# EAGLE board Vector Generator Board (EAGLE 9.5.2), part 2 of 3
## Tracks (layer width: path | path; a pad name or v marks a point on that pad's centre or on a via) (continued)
DX2 (continued)
  Bottom 0.381: 3A.6 77.67,269.48 81.18,272.99 93.15,272.99 96.95,269.19 98.7,269.19 99.58,270.07 99.58,275.32 97.83,275.32 4A.3
DX3
  Bottom 0.381: 4A.4 97.54,273.28 90.23,280.58 78.84,280.58 77.67,279.41 3A.2
DX4
  Bottom 0.381: 4A.5 97.54,270.65 89.06,279.12 85.27,279.12 3A.15
DX5  (via drill 0.35)
  Top 0.381: v87.02,243.19 87.02,230.63 85.27,228.88 3B.9
  Bottom 0.381: v87.02,243.19 87.31,242.9 97.24,242.9 97.54,242.61 4B.2
DX6
  Bottom 0.381: 3B.6 77.67,233.84 78.26,234.43 80.89,234.43 83.81,237.35 93.15,237.35 96.66,233.84 99,233.84 100.17,235.01 100.17,239.98 97.83,239.98 4B.3
DX7
  Bottom 0.381: 3B.2 77.67,243.78 81.47,239.98 92.28,239.98 94.62,237.64 97.54,237.64 4B.4
DX8
  Bottom 0.381: 4B.5 97.83,235.01 99.58,236.77 99.58,238.81 94.32,238.81 90.82,242.32 86.73,242.32 85.27,243.78 3B.15
DX9  (via drill 0.35)
  Top 0.381: v89.65,207.26 v89.65,193.24
  Bottom 0.381: v89.65,193.24 85.27,193.24 3C.9 | v89.65,207.26 97.54,207.26 4C.2
DX10  (via drill 0.35)
  Top 0.381: v90.23,191.49 94.03,195.29 94.03,202.01 96.37,204.34 97.54,204.34 4C.3
  Bottom 0.381: 3C.6 84.1,191.49 v90.23,191.49
DX11  (via drill 0.35)
  Top 0.381: v95.78,199.96 97.54,201.71 4C.4
  Bottom 0.381: v95.78,199.96 91.11,204.63 83.81,204.63 80.89,207.56 78.26,207.56 77.67,208.14 3C.2
DX12
  Bottom 0.381: 4C.5 97.54,199.67 91.4,205.8 87.61,205.8 85.27,208.14 3C.15
DY1
  Top 0.381: 3D.9 85.27,157.61 89.06,157.61 89.06,162.87 97.54,171.34 4D.2
DY2
  Bottom 0.381: 3D.6 77.67,162.57 78.55,163.45 81.18,163.45 84.1,166.37 90.82,166.37 94.62,162.57 98.7,162.57 99.58,163.45 99.58,168.71 97.83,168.71 4D.3
DY3  (via drill 0.35)
  Top 0.381: v81.47,173.97 80.3,172.8 77.67,172.8 3D.2
  Bottom 0.381: v81.47,173.97 89.94,173.97 97.54,166.37 4D.4
DY4
  Bottom 0.381: 4D.5 97.54,164.03 94.91,166.66 91.4,166.66 85.56,172.5 85.27,172.5 3D.15
DY5
  Top 0.381: 3E.9 85.27,121.97 87.9,124.6 99.58,124.6 99.58,133.95 97.83,135.7 4E.2
DY6
  Top 0.381: 3E.6 77.67,127.23 79.43,127.23 80.01,127.81 80.89,127.81 82.93,125.77 96.08,125.77 96.08,131.61 97.54,133.07 4E.3
DY7  (via drill 0.35)
  Top 0.381: v92.28,131.32 92.28,131.03 83.81,131.03 82.06,132.78 82.06,136.28 78.55,136.28 77.67,137.16 3E.2
  Bottom 0.381: v92.28,131.32 92.57,131.03 97.54,131.03 4E.4
DY8
  Bottom 0.381: 4E.5 97.54,128.4 95.49,130.44 91.99,130.44 85.27,137.16 3E.15
DY9
  Top 0.381: 3F.9 85.27,86.63 95.2,96.56 99.58,96.56 99.58,98.31 97.83,100.06 4F.2
DY10
  Top 0.381: 3F.6 77.67,91.59 78.55,91.59 79.13,92.18 80.01,92.18 80.01,95.1 82.64,97.73 97.54,97.73 4F.3
DY11
  Bottom 0.381: 4F.4 97.54,95.39 87.61,105.32 76.21,105.32 75.63,104.74 75.63,101.82 77.38,101.82 3F.2
DY12
  Bottom 0.381: 4F.5 97.54,92.76 88.77,101.52 85.27,101.52 3F.15
FRAMECOMPLETE  (via drill 0.35)
  Top 0.381: v4.94,113.21 4.94,114.67 P1.20 | v46.42,27.04 v46.42,43.1 46.42,48.95 44.67,50.7 1G.12 | v96.08,43.4 96.08,55.66 97.54,57.12 4G.5 97.83,57.42 100.17,59.75 100.17,61.51 102.79,64.14 102.79,110 v102.21,110.58 | v24.8,114.38 31.23,114.38 v31.23,112.92
  Bottom 0.381: v4.94,113.21 4.94,114.38 | 4.94,114.38 4.94,114.67 P1.20 4.94,114.38 | v46.42,27.04 46.42,26.45 45.54,25.58 40.87,25.58 37.07,21.78 1H.5 | v96.08,43.4 95.49,42.81 46.71,42.81 v46.42,43.1 | v24.8,114.38 4.94,114.38 | v31.23,112.92 31.52,112.62 67.45,112.62 69.49,110.58 v102.21,110.58
GND  (via drill 0.35, 0.8)
  Top 0.381: IC13.13 157.71,45.44 161.21,41.94 161.21,35.8 R47.2 | C44.2 162.67,19.15 169.98,26.45 169.98,36.68 C48.2 | IC8.13 157.71,106.49 161.21,102.98 161.21,96.56 R34.2 | C45.2 181.66,62.38 188.96,69.69 188.96,79.91 C40.2 | v161.51,90.13 161.51,81.08 162.38,80.2 C28.2 | C34.2 209.41,110.58 202.11,117.88 200.94,117.88 R41.2 | C35.2 166.47,124.6 172.61,124.6 C36.2 | 238.33,94.22 241.25,97.14 X1.4 | 238.33,94.22 238.33,92.47 241.25,89.55 X1.2 | 238.33,94.22 238.33,102.11 241.25,105.03 X1.6 | R54.2 200.94,54.5 207.07,48.36 209.41,48.36 C50.2 | 219.63,65.89 218.47,67.06 C53.2 218.17,67.35 216.13,67.35 212.92,70.56 212.92,93.64 213.21,93.93 C41.2 | 219.63,65.89 219.63,48.36 218.47,47.19 C54.2 218.47,46.9 218.47,42.52 215.54,39.6 215.54,31.42 214.67,30.54 C57.2 | 219.63,65.89 219.63,81.08 223.43,84.87 C42.2 | C1.2 186.92,162.57 187.8,163.45 187.8,168.71 X2.2 | R26.1 142.52,170.46 142.52,169 R23.1 | C27.2 147.48,157.61 147.48,163.74 Q1.1 | C5.- 230.15,138.62 232.19,140.67 232.19,143.29 IC1.GND | C6.- 210.87,138.62 213.21,140.96 213.21,143.29 IC2.GND | 228.4,128.27 228.4,116.13 224.02,116.13 218.47,110.58 C38.2 218.17,110.29 218.17,107.66 v216.13,105.61 | D6.C 147.19,143.59 147.19,149.72 C8.2 | C7.+ 155.08,137.16 155.08,143.29 IC3.GND | 8A.4 179.32,274.45 180.78,275.91 180.78,277.66 179.32,279.12 8A.2 | 9A.2 199.48,279.12 201.23,277.37 201.23,276.2 199.48,274.45 9A.4 199.19,274.15 197.43,272.4 197.43,265.98 199.19,264.22 9A.8 | 3H.4 77.38,25.29 77.38,22.95 3H.5 77.38,22.66 75.63,20.9 75.63,17.11 77.38,15.35 3H.8 | 4H.19 4H.18 | 1G.1 37.07,71.14 37.36,71.44 37.36,83.41 37.07,83.71 1F.10
  Top 0.381: 2F.1 57.23,106.78 57.23,123.14 2E.7 | 2D.1 57.23,178.05 57.23,194.12 2C.7 | 4D.1 97.83,174.26 97.83,194.12 4C.7 | 2B.1 57.23,249.03 57.23,265.39 2A.7 | 4A.1 97.83,280.58 99.58,278.83 99.58,267.44 97.83,265.68 4A.7 | LED2.K 219.93,167.83 219.93,194.12 10C.7 | T1.3 139.6,167.83 139.31,168.12 139.31,193.24 138.43,194.12 6C.7
  Top 1.016: D5.A D7.A C9.2 228.4,128.27 C10.2
  Top 2.54: P1.21 4.83,109.47 v5.08,109.22 5.08,107.24 P1.22
  Bottom 0.381: C56.2 188.96,15.35 184.29,15.35 R50.1 184,15.35 183.71,15.65 165.89,15.65 162.67,18.86 C44.2 | C46.2 144.86,27.92 149.82,27.92 IC12.1 150.11,28.21 157.42,35.51 161.21,35.51 R47.2 161.51,35.8 162.38,36.68 169.98,36.68 C48.2 | C30.2 144.86,88.96 149.82,88.96 IC7.1 150.11,88.96 151.28,90.13 | C32.2 169.98,97.73 162.67,97.73 161.51,96.56 R34.2 161.21,96.27 157.42,96.27 151.28,90.13 | 177.57,62.09 176.69,61.21 R52.1 | 177.57,62.09 181.37,62.09 C45.2 181.66,62.09 188.09,55.66 199.77,55.66 200.65,54.79 R54.2 | 177.57,62.09 176.4,63.26 172.9,63.26 C52.2 172.61,63.55 166.47,63.55 C51.2 166.18,63.26 159.75,63.26 157.71,61.21 IC13.19 157.42,60.92 155.66,60.92 155.66,47.48 157.42,45.73 IC13.13 | 185.46,79.91 184.29,78.74 R37.1 | 185.46,79.91 188.96,79.91 C40.2 | 185.46,79.91 162.67,79.91 C28.2 | v161.51,90.13 151.28,90.13 | IC8.19 157.71,121.97 160.05,124.31 166.18,124.31 C35.2 | 177.86,123.14 176.69,121.97 R39.1 | 177.86,123.14 181.37,123.14 C29.2 185.46,119.34 199.48,119.34 200.65,118.17 R41.2 | 177.86,123.14 174.07,123.14 172.9,124.31 C36.2 | C42.2 223.72,85.17 227.52,88.96 240.96,88.96 241.25,89.26 X1.2 | C57.2 214.38,30.25 213.5,29.38 207.07,29.38 203.28,25.58 C55.2 203.28,25.29 221.09,25.29 C58.2 | C39.2 202.11,88.96 205.91,92.76 212.04,92.76 213.21,93.93 C41.2 213.21,94.22 213.21,105.61 | C54.2 218.17,47.19 217.88,47.48 214.38,47.48 213.79,48.07 209.7,48.07 C50.2 | 213.21,105.61 213.21,106.78 209.7,110.29 C34.2 | C1.2 186.92,162.57 188.96,162.57 C2.2 | R23.1 142.23,168.71 140.77,168.71 T1.3 139.89,167.54 147.78,167.54 148.95,166.37 | 148.95,166.37 LED4.A 161.51,166.37 162.09,165.79 184.87,165.79 187.8,168.71 X2.2
  Bottom 0.381: 148.95,166.37 147.48,164.91 147.48,164.03 Q1.1 | 219.63,129.56 220.8,128.4 224.6,128.4 C10.2 | 219.63,129.56 218.47,130.73 C37.2 218.47,131.03 221.97,134.53 226.06,134.53 229.86,138.33 C5.- | 219.63,129.56 212.04,129.56 212.04,137.16 210.87,138.33 C6.- | 152.74,145.63 149.53,145.63 147.48,143.59 D6.C | 152.74,145.63 154.79,143.59 IC3.GND | 168.52,145.63 168.81,145.92 C4.+ 168.52,145.63 | 152.74,145.63 168.52,145.63 | 188.96,143.29 191.59,145.92 C3.- | 188.96,143.29 170.85,143.29 168.52,145.63 | 188.96,143.29 197.73,143.29 199.48,141.54 211.46,141.54 213.21,143.29 IC2.GND | C27.2 147.48,157.31 147.48,150.01 C8.2 | 8A.2 179.32,279.12 180.2,278.24 198.31,278.24 199.19,279.12 9A.2 | 75.63,26.75 75.63,25.58 77.38,25.58 3H.4 | 75.63,26.75 75.63,31.13 77.38,32.88 3H.1 | 75.63,26.75 78.55,26.75 81.76,29.96 84.68,29.96 84.98,30.25 3H.15 | LED2.K 219.93,167.83 224.6,167.83 LED1.K | 27.94,112.04 34.73,112.04 34.73,110.87 34.44,110.58 34.44,108.83 35.03,108.24 35.32,108.24 36.78,106.78 1F.1 | 27.94,177.76 36.78,177.76 1D.1 | 27.94,213.4 36.78,213.4 1C.1 | 27.94,249.03 36.78,249.03 1B.1 | LED3.K 231.03,222.45 224.02,222.45 C15.2 | 4H.18 109.22,22.66 116.23,15.65 117.98,15.65 5H.8 | v216.13,105.61 213.21,105.61
  Bottom 1.016: 3H.8 77.47,8.89 | 77.47,8.89 77.47,8.74 85.09,8.74 | 85.09,8.74 93.98,8.74 | 85.09,8.74 3H.9 3H.10 | 5H.8 118.11,8.89 117.96,8.74 93.98,8.74 | 4H.12 93.98,8.74 | 27.94,46.84 36.83,46.84 | 36.83,46.84 1G.10 | 36.83,46.84 57.15,46.84 | 57.15,46.84 77.32,46.84 | 3G.7 77.47,46.99 77.32,46.84 | 77.32,46.84 97.64,46.84 | 4G.7 97.79,46.99 97.64,46.84 | 97.64,46.84 117.96,46.84 118.11,46.99 5G.8 | 27.94,80.01 36.83,80.01 | 36.83,80.01 C17.2 57.15,80.01 | 57.15,80.01 C19.2 C21.2 92.71,80.01 | 92.71,80.01 C23.2 118.11,80.01 | 118.11,80.01 C25.2 | 2F.10 57.15,80.01 | 3F.12 86.36,93.98 92.71,87.63 | 92.71,87.63 92.71,80.01 | 92.71,87.63 4F.7 | 5F.8 118.11,80.01 | 27.94,119.38 36.83,119.38 | 36.83,119.38 57.15,119.38 | 36.83,119.38 1E.7 | 2E.7 57.15,119.38 | 57.15,119.38 91.44,119.38 | 3E.12 86.36,129.54 91.44,124.46 91.44,123.19 | 91.44,123.19 91.44,119.38 | 91.44,123.19 4E.7 | 91.44,119.38 118.11,119.38 5E.8 | 77.47,8.89 57.15,8.89 | 57.15,8.89 36.83,8.89 | 36.83,8.89 27.94,8.89 | 36.83,8.89 1H.7 | 2H.7 57.15,8.89 | 27.94,152.4 36.83,152.4 | 36.83,152.4 57.15,152.4 | 57.15,152.4 91.44,152.4 | 91.44,152.4 118.11,152.4 5D.8 | 3D.12 86.36,165.1 91.44,160.02 91.44,158.75 | 91.44,158.75 91.44,152.4 | 91.44,158.75 4D.7 | 2D.10 57.15,152.4 | 27.94,187.96 36.83,187.96 | 36.83,187.96 57.15,187.96 | 57.15,187.96 91.44,187.96 | 91.44,187.96 118.11,187.96 | 118.11,187.96 128.27,187.96 130.81,190.5 138.43,190.5 | 138.43,190.5 158.75,190.5 | 158.75,190.5 179.07,190.5 | 179.07,190.5 199.39,190.5 | 199.39,190.5 219.71,190.5 10C.7 | 9C.8 199.39,190.5 | 179.07,190.5 8C.8 | 7C.7 158.75,190.5 | 138.43,190.5 6C.7 | 5C.8 118.11,187.96 | 3C.12 86.36,200.66 91.44,195.58 91.44,194.31 | 91.44,194.31 91.44,187.96
  Bottom 1.016: 91.44,194.31 4C.7 | 2C.7 57.15,187.96 | 1C.10 36.83,187.96 | 27.94,220.98 29.21,222.25 36.83,222.25 | 36.83,222.25 C12.2 57.15,222.25 | 57.15,222.25 C14.2 C16.2 91.44,222.25 | 91.44,222.25 C18.2 118.11,222.25 | 118.11,222.25 C20.2 138.43,222.25 | 138.43,222.25 C22.2 158.75,222.25 | 158.75,222.25 C24.2 179.07,222.25 | 179.07,222.25 C11.2 199.39,222.25 | 199.39,222.25 C13.2 C15.2 | 9B.8 199.39,222.25 | 179.07,222.25 8B.8 | 158.75,222.25 7B.7 | 138.43,222.25 6B.8 | 118.11,222.25 5B.8 | 3B.12 86.36,236.22 91.44,231.14 91.44,229.87 | 91.44,229.87 91.44,222.25 | 91.44,229.87 4B.7 | 2B.10 57.15,222.25 | 1B.10 36.83,222.25 | 27.94,260.35 36.83,260.35 | 36.83,260.35 57.15,260.35 | 57.15,260.35 91.44,260.35 | 91.44,260.35 118.11,260.35 | 118.11,260.35 138.43,260.35 | 138.43,260.35 158.75,260.35 | 158.75,260.35 179.07,260.35 | 179.07,260.35 199.39,260.35 9A.8 | 8A.8 179.07,260.35 | 158.75,260.35 7A.7 | 6A.8 138.43,260.35 | 5A.8 118.11,260.35 | 3A.12 86.36,271.78 91.44,266.7 91.44,265.43 | 91.44,265.43 91.44,260.35 | 91.44,265.43 4A.7 | 2A.7 57.15,260.35 | 1A.7 36.83,260.35 | 2G.7 57.15,46.84 | 36.83,152.4 1D.10 | 1F.10 36.83,80.01
  Bottom 2.54: P1.21 4.83,109.22 P1.22 | X3.2 15.95,285.75 27.94,273.76 27.94,260.35
  Bottom 5.08: 4.83,109.22 v5.08,109.22 27.94,109.22 | 27.94,260.35 27.94,249.03 27.94,220.98 27.94,213.4 27.94,187.96 27.94,177.76 27.94,152.4 27.94,119.38 27.94,112.04 27.94,109.22 | 27.94,109.22 27.94,80.01 27.94,46.84 27.94,8.89
  pour Top: 247.65,0 133.35,0 133.35,142.24 133.35,143.51 129.54,147.32 129.54,187.96 247.65,187.96
  pour Bottom (isolate 0.254): 247.65,0 133.35,0 133.35,143.51 128.27,148.59 128.27,187.96 247.65,187.96
HALTROTATE  (via drill 0.35)
  Top 0.381: v49.05,23.83 49.34,24.12 v49.34,43.69 | v94.32,64.72 v94.32,43.69
  Bottom 0.381: v49.05,23.83 47.3,22.07 44.96,22.07 44.67,21.78 1H.10 | v49.34,43.69 49.63,43.4 94.03,43.4 v94.32,43.69 | v94.32,64.72 97.54,64.72 4G.2
INHIBITX  (via drill 0.35)
  Top 0.381: v43.2,139.79 43.79,140.37 v43.79,153.52 | v47.3,184.77 v47.3,153.52 | v160.63,180.68 160.92,180.97 160.92,191.49 166.18,196.75 7C.9
  Bottom 0.381: v43.2,139.79 38.24,139.79 37.07,138.62 1E.1 | v47.3,153.52 v43.79,153.52 | v47.3,184.77 48.46,185.94 73.29,185.94 75.04,184.19 82.64,184.19 83.22,184.77 105.72,184.77 108.64,181.85 129.08,181.85 130.25,180.68 v160.63,180.68 | 8C.6 179.03,197.92 178.45,197.33 166.76,197.33 166.47,197.04 7C.9
INHIBITY  (via drill 0.35)
  Top 0.381: v71.83,159.65 v71.83,145.05 | v74.46,185.94 v74.46,160.82 | v110.68,185.94 110.97,186.23 110.97,199.38 111.27,199.67 v111.27,219.82 | v158.59,219.82 158.59,209.6 7C.1
  Bottom 0.381: v71.83,145.05 46.13,145.05 45.83,145.34 37.07,145.34 34.44,142.71 33.27,142.71 33.27,136.87 33.86,136.28 36.49,136.28 36.78,135.99 1E.2 | v71.83,159.65 73,160.82 v74.46,160.82 | v110.68,185.94 v74.46,185.94 | v158.59,219.82 v111.27,219.82 | 9C.6 199.19,198.21 197.73,199.67 192.47,199.67 187.5,204.63 168.52,204.63 167.35,205.8 164.43,205.8 160.92,209.31 158.88,209.31 7C.1
INTENSITY0  (via drill 0.35)
  Top 0.381: v42.62,82.25 42.62,70.56 44.37,68.81 1G.19 | v49.63,82.54 49.92,82.83 49.92,128.4 v49.63,128.69 | v53.72,128.69 54.01,128.98 54.01,148.55 53.43,149.14 53.43,150.31 54.01,150.89 54.01,163.74 v53.72,164.03 | v59.86,164.03 60.73,164.91 v60.73,186.82 | 7A.1 158.88,280.58 160.05,279.41 174.07,279.41 174.07,184.19 R20.1
  Bottom 0.381: v42.62,82.25 42.91,82.54 v49.63,82.54 | v53.72,128.69 v49.63,128.69 | v59.86,164.03 v53.72,164.03 | v60.73,186.82 112.43,186.82 115.94,183.31 133.46,183.31 134.34,184.19 148.65,184.19 150.7,182.14 172.02,182.14 173.77,183.9 R20.1
INTENSITY1  (via drill 0.35)
  Top 0.381: v53.72,66.18 53.72,83.71 53.14,84.29 v53.14,90.13 | v58.98,90.13 59.56,90.72 59.56,93.64 62.19,96.27 62.19,98.9 63.65,100.36 66.57,100.36 v66.57,115.55 | v99,120.8 v99,115.55 | v110.39,120.8 110.1,121.09 110.1,138.62 110.39,138.91 110.39,143.88 v110.1,144.17 | v196.85,140.67 197.14,140.96 197.14,153.22 202.69,158.78 202.69,182.44 201.52,183.6 v201.52,184.77 | v173.19,277.08 173.19,187.11 170.27,184.19 R19.1
  Bottom 0.381: v53.72,66.18 44.67,66.18 1G.18 | v58.98,90.13 v53.14,90.13 | v99,115.55 v66.57,115.55 | v110.39,120.8 v99,120.8 | v110.1,144.17 123.53,144.17 123.83,144.46 132,144.46 135.51,140.96 196.56,140.96 v196.85,140.67 | v201.52,184.77 174.94,184.77 174.36,185.36 171.44,185.36 170.27,184.19 R19.1 | v173.19,277.08 159.75,277.08 158.88,277.95 7A.2
INTENSITY2  (via drill 0.35)
  Top 0.381: v58.1,68.81 58.39,69.1 v58.39,81.66 | v91.4,81.66 96.08,86.34 96.08,88.09 96.95,88.96 99.58,88.96 99.58,91.01 100.17,91.59 100.17,115.84 99.87,116.13 99.87,124.02 100.46,124.6 v100.46,126.94 | v94.32,154.39 v94.32,128.11 | v116.81,154.39 117.4,153.81 v117.4,148.84 | v150.41,148.84 150.41,158.19 157.42,165.2 157.42,171.63 161.51,175.72 161.51,185.94 165.01,189.45 166.18,189.45 | 166.18,189.45 166.18,184.19 R18.1 | 166.18,189.45 168.81,192.07 168.81,223.04 164.43,227.42 164.43,276.2 166.18,277.95 7A.13
  Bottom 0.381: v58.1,68.81 55.18,68.81 55.18,66.47 54.01,65.3 46.42,65.3 44.67,63.55 1G.17 | v91.4,81.66 v58.39,81.66 | v100.46,126.94 95.49,126.94 v94.32,128.11 | v116.81,154.39 v94.32,154.39 | v117.4,148.84 117.69,149.14 141.35,149.14 141.94,148.55 148.95,148.55 149.24,148.84 v150.41,148.84
INTENSITY3  (via drill 0.35)
  Top 0.381: v93.45,78.74 v93.45,63.55 | v146.32,78.74 147.78,80.2 v148.07,80.2 | v173.48,81.08 173.77,81.37 173.77,104.15 172.9,105.03 172.9,123.14 173.77,124.02 173.77,126.94 173.48,127.23 v173.48,128.4 | v174.07,157.61 v174.07,135.41 | v164.43,163.74 164.43,182.14 162.67,183.9 R17.1 | v154.5,203.47 154.5,204.63 155.66,205.8 155.66,269.19 159.75,269.19 160.63,270.07 160.63,273.57 158.88,275.32 7A.3 | v149.82,200.25 149.82,183.9 150.7,183.02 151.87,183.02 151.87,183.31 154.5,185.94 157.42,185.94 v157.42,185.06
  Bottom 0.381: v93.45,63.55 56.06,63.55 54.31,61.8 45.25,61.8 44.67,61.21 1G.16 | v93.45,78.74 113.02,78.74 113.31,79.03 121.2,79.03 121.49,78.74 v146.32,78.74 | v148.07,80.2 161.21,80.2 162.09,81.08 v173.48,81.08 | v173.48,128.4 174.07,128.98 v174.07,135.41 | v174.07,157.61 174.07,158.19 173.77,158.48 173.77,161.99 174.36,162.57 174.36,163.74 v164.43,163.74 | v154.5,203.47 151.28,200.25 v149.82,200.25 | v157.42,185.06 157.71,185.36 161.21,185.36 162.38,184.19 R17.1
INTENSITY4  (via drill 0.35)
  Top 0.381: v51.09,58.59 51.09,147.09 v51.38,147.38 | v153.62,163.45 153.62,171.63 157.42,175.43 157.42,182.73 158.59,183.9 R16.1 | v153.33,203.47 153.33,270.36 155.96,270.36 158.59,272.99 7A.4 | v148.95,200.84 148.95,183.9 150.41,182.44 152.74,182.44 v152.74,183.02
  Bottom 0.381: v51.09,58.59 44.67,58.59 1G.15 | v51.38,147.38 51.68,147.09 114.19,147.09 116.81,149.72 137.85,149.72 151.57,163.45 v153.62,163.45 | v153.33,203.47 150.99,201.13 149.24,201.13 v148.95,200.84 | v152.74,183.02 157.71,183.02 158.59,183.9 R16.1
INTENSITY5  (via drill 0.35)
  Top 0.381: v46.42,6.59 46.42,25.29 43.5,25.29 42.62,26.16 42.62,53.91 44.37,55.66 1G.14 | v174.65,34.34 v174.65,6.59 | v182.83,34.34 182.83,59.46 180.49,61.8 180.49,62.67 185.46,67.64 186.04,67.64 187.8,69.39 187.8,85.17 185.46,87.5 185.46,114.08 191.01,119.63 v191.01,132.19 | v188.96,151.18 v188.96,133.36 | v200.65,151.47 203.28,154.1 203.28,182.73 202.4,183.6 v202.4,185.94 201.52,186.82 v201.52,218.36 | v154.79,218.36 154.79,269.77 156.25,269.77 156.83,270.36 158.59,270.36 7A.5
  Bottom 0.381: v174.65,6.59 v46.42,6.59 | v182.83,34.34 v174.65,34.34 | v191.01,132.19 189.84,133.36 v188.96,133.36 | v188.96,151.18 189.25,151.47 v200.65,151.47 | v202.4,185.94 201.82,186.53 156.54,186.53 155.08,185.06 155.08,184.19 R15.1 | v201.52,218.36 v154.79,218.36
INTENSITY6  (via drill 0.35)
  Top 0.381: v47.3,78.45 47,78.16 47,73.19 47.3,72.9 47.3,56.25 44.67,53.62 1G.13 | v113.6,78.16 113.89,78.45 113.89,93.34 113.6,93.64 113.6,126.94 114.19,127.52 v114.19,129.86 | v129.08,133.36 128.79,133.66 128.79,169.58 129.38,170.17 129.38,170.75 128.79,171.34 128.79,183.31 v131.13,185.65 | v164.43,197.33 160.05,192.95 151.28,192.95 151.28,184.19 R14.1
  Bottom 0.381: v47.3,78.45 92.57,78.45 93.15,77.86 113.31,77.86 v113.6,78.16 | v114.19,129.86 116.23,131.9 116.23,135.7 122.37,135.7 124.7,133.36 v129.08,133.36 | v131.13,185.65 131.42,185.36 149.82,185.36 150.99,184.19 R14.1 | v164.43,197.33 164.43,199.96 166.18,201.71 7C.11
INVX
  Top 0.381: Q3.1 223.43,93.93 221.09,91.59 221.09,90.42 R59.2
  Bottom 0.381: IC11.13 216.13,85.17 218.17,87.21 218.17,90.13 R61.2 218.47,90.13 220.8,90.13 R59.2
INVY
  Top 0.381: IC16.13 217.3,21.78 220.8,25.29 220.8,27.92 R62.2 | Q4.1 226.06,31.71 223.72,29.38 223.72,28.21 R60.2
  Bottom 0.381: R60.2 223.43,27.92 221.09,27.92 R62.2
LDX2  (via drill 0.35)
  Top 0.381: v48.46,190.61 48.17,190.91 48.17,222.45 44.67,225.96 1B.11 | v34.44,20.32 34.44,39.31 38.82,43.69 38.82,71.44 38.24,72.02 38.24,82.83 38.82,83.41 v38.82,88.09 | v42.62,114.08 v42.62,88.09 | v35.03,114.08 35.03,139.2 40.58,144.75 40.58,186.53 44.37,190.32 1C.11
  Bottom 0.381: v48.46,190.61 44.67,190.61 1C.11 | v34.44,20.32 37.95,20.32 40.28,22.66 45.25,22.66 48.17,25.58 49.34,25.58 54.6,20.32 58.1,20.32 61.02,17.4 63.65,17.4 64.53,16.52 2H.8 | v42.62,88.09 v38.82,88.09 | v35.03,114.08 v42.62,114.08
LDXY1  (via drill 0.35)
  Top 0.381: v61.9,159.36 62.19,159.65 62.19,162.28 63.94,164.03 66.57,164.03 66.57,165.49 65.7,166.37 61.9,166.37 61.9,215.74 64.53,218.36 64.53,225.96 2B.11 | v48.46,73.77 v48.46,24.7 | v63.65,73.77 64.53,74.65 64.53,83.71 2F.11 | v66.57,131.61 66.57,152.93 64.82,154.69 2D.11 | v60.44,127.81 60.73,127.52 v60.73,95.97 | v69.2,84 v69.2,95.1
  Bottom 0.381: v61.9,159.36 61.9,156.73 62.48,156.15 63.36,156.15 64.53,154.98 2D.11 | v48.46,24.7 49.34,24.7 54.31,19.74 56.35,19.74 56.93,19.15 2H.6 | v63.65,73.77 v48.46,73.77 | v66.57,131.61 66.57,129.56 62.19,129.56 v60.44,127.81 | v60.73,95.97 61.61,95.1 v69.2,95.1 | v69.2,84 64.82,84 2F.11
LDY2  (via drill 0.35)
  Top 0.381: v40.28,84 40.28,86.63 40.58,86.92 40.58,117.59 40.28,117.88 40.28,131.61 43.5,134.82 45.83,134.82 45.83,135.12 46.42,135.7 46.42,144.75 44.67,146.51 44.67,154.69 1D.11 | v55.18,40.77 55.18,26.16 56.93,24.41 2H.4 | v47.59,40.77 47.88,41.06 47.88,73.19 47.59,73.48 47.59,77.57 48.17,78.16 48.17,80.2 44.67,83.71 1F.11
  Bottom 0.381: v40.28,84 44.37,84 1F.11 | v47.59,40.77 v55.18,40.77
LDZ
  Bottom 0.381: 1G.11 44.67,48.36 54.89,58.59 101.62,58.59 105.13,62.09 4G.12
N$1
  Top 1.016: IC3.IN 152.4,151.13 160.02,158.75 D3.A 179.07,154.94 C4.- 185.42,152.4 194.31,152.4 D4.A
N$2  (via drill 0.35)
  Top 0.381: v38.82,4.84 38.82,17.11 37.07,18.86 1H.6 | v243,30.54 v243,4.84 | v241.25,32 241.25,63.55 R25.1
  Bottom 0.381: v243,4.84 v38.82,4.84 | v243,30.54 241.54,32 v241.25,32
N$3  (via drill 0.35)
  Top 0.381: v41.75,78.74 v41.75,30.54 | v33.27,105.61 v33.27,78.74 | v48.46,105.61 48.75,105.91 48.75,113.79 48.17,114.38 48.17,126.64 48.75,127.23 v48.75,130.73
  Bottom 0.381: v41.75,30.54 35.03,30.54 35.03,26.16 36.78,24.41 1H.4 | v33.27,78.74 v41.75,78.74 | v48.46,105.61 v33.27,105.61 | v48.75,130.73 44.67,130.73 1E.11
N$4  (via drill 0.35)
  Top 0.381: R23.2 155.08,169 155.08,171.34 R15.2 | v133.46,154.98 133.46,147.38 R22.1 | R14.2 150.99,171.34 149.24,169.58 149.24,165.2 Q1.2
  Bottom 0.381: R20.2 173.77,171.63 170.27,171.63 R19.2 169.98,171.63 166.47,171.63 R18.2 166.18,171.63 162.67,171.63 R17.2 162.38,171.63 158.88,171.63 R16.2 158.59,171.63 155.08,171.63 R15.2 154.79,171.63 151.28,171.63 R14.2 | v133.46,154.98 134.63,156.15 142.52,156.15 148.95,162.57 148.95,164.91 Q1.2
N$5
  Top 0.381: Q2.2 236.28,54.2 236.28,55.66 R25.2
  Bottom 0.381: R27.1 232.49,55.96 235.99,55.96 R25.2
N$6
  Top 1.016: R7.1 LED1.A
N$8
  Top 1.016: LED2.A 220.98,163.83 R8.1
N$9
  Top 0.381: R9.1 231.32,217.19 231.32,219.53 LED3.A
N$10
  Bottom 0.381: R44.2 191.88,50.99 198.02,50.99 VR3.3
N$11  (via drill 0.35)
  Top 0.381: R38.1 171.73,93.93 172.61,93.05 172.61,88.96 R29.1 | R36.1 218.17,126.94 217.3,126.06 v217.3,123.14 217.3,107.95 215.25,105.91 215.25,94.22 213.5,92.47 213.5,74.94 215.84,72.61 IC11.8 215.84,72.31 v215.84,68.81
  Bottom 0.381: v217.3,123.14 213.5,123.14 IC10.7 | C31.1 227.23,123.43 223.72,126.94 218.47,126.94 R36.1 | v215.84,68.81 215.54,69.1 208.83,69.1 191.59,86.34 175.24,86.34 172.9,88.67 R29.1
N$12
  Top 0.381: C27.1 142.23,157.61 139.89,159.94 139.89,164.91 T1.1 139.6,165.2 138.72,165.2 137.55,166.37 R24.1
  Bottom 0.381: R24.1 T2.2 | T1.1 139.89,165.2 146.03,165.2 147.19,166.37 Q1.3
N$13
  Bottom 0.381: IC7.16 157.71,88.96 159.75,88.96 R29.2
N$14
  Top 0.381: T1.2 141.35,166.37 141.06,166.66 141.06,175.13 142.23,176.3 C26.2 142.52,176.59 142.52,178.05 147.19,182.73 R21.1
N$15  (via drill 0.35)
  Top 0.381: v108.64,57.42 108.64,66.47 107.17,67.93 107.17,112.04 107.76,112.62 111.27,112.62 112.43,113.79 112.43,129.86 v112.73,130.15 | v113.02,131.9 112.73,132.19 112.73,153.81 110.1,156.44 110.1,176.89 v110.39,177.18 | R21.2 134.63,182.73 136.97,180.39 136.97,176.59 C26.1
  Bottom 0.381: v108.64,57.42 105.42,57.42 4G.10 | v112.73,130.15 112.73,131.9 v113.02,131.9 | v110.39,177.18 110.97,176.59 122.07,176.59 124.7,173.97 134.63,173.97 136.97,176.3 C26.1
N$16
  Top 0.381: IC11.3 208.53,82.83 210,84.29 210,86.04 208.53,87.5 IC11.1 208.24,87.8 208.24,93.93 C41.1
N$17
  Top 0.381: IC11.9 215.84,74.94 214.08,76.69 214.08,78.16 215.84,79.91 IC11.11
  Bottom 0.381: C42.1 223.43,80.2 216.13,80.2 IC11.11
N$18
  Bottom 0.381: IC11.10 215.84,77.57 208.53,84.87 IC11.2 208.53,85.17 212.33,88.96 217,88.96 217,116.13 213.79,119.34 207.07,119.34 205.91,120.51 IC10.3
N$19
  Top 0.381: R40.1 184.29,101.52 184.29,94.22 R38.2
  Bottom 0.381: R38.2 184.29,93.93 186.63,93.93 IC9.2
N$20
  Bottom 0.381: R37.2 184.29,91.59 186.63,91.59 IC9.3
N$21
  Bottom 0.381: 196.85,91.3 194.51,91.3 IC9.6 | 196.85,91.3 197.14,91.3 208.24,80.2 IC11.4 | 196.85,91.3 R40.2
N$22
  Bottom 0.381: IC13.1 149.82,63.55 144.86,63.55 JP4.1
N$23
  Top 0.381: R41.1 188.09,118.17 188.09,120.51 C43.2
  Bottom 0.381: IC10.2 205.61,123.14 198.31,123.14 VR2.1 198.02,123.14 190.42,123.14 188.09,120.8 C43.2
N$24
  Bottom 0.381: IC13.2 149.82,60.92 144.86,60.92 JP4.2
N$25  (via drill 0.35)
  Top 0.381: R51.1 171.73,30.25 171.73,29.08 172.61,28.21 R42.1 172.9,27.92 173.77,27.04 v173.77,10.68 | IC16.8 217,8.93 213.5,12.43 213.5,38.43 217.88,42.81 217.88,46.02 217.3,46.61 217.3,62.38 218.17,63.26 R49.1
  Bottom 0.381: 218.47,59.75 224.6,59.75 C47.1 | 218.47,59.75 213.5,59.75 IC15.7 | v173.77,10.68 176.69,7.76 216.13,7.76 217,8.64 IC16.8 | 218.47,59.75 218.47,63.26 R49.1
N$26
  Bottom 0.381: IC12.16 157.71,27.92 159.75,27.92 R42.2
N$27
  Top 0.381: IC16.3 209.7,19.15 211.46,20.9 211.46,22.37 209.7,24.12 IC16.1 209.7,24.41 209.7,30.25 C57.1
N$28
  Top 0.381: IC16.9 219.05,13.31 219.05,14.48 217.3,16.23 IC16.11
  Bottom 0.381: C58.1 224.6,16.52 217.3,16.52 IC16.11
N$29  (via drill 0.35)
  Top 0.381: v217,45.73 217,42.81 207.66,33.46 207.66,23.53 209.41,21.78 IC16.2
  Bottom 0.381: IC16.2 209.7,21.49 217,14.19 IC16.10 | v217,45.73 219.63,45.73 219.63,47.48 219.05,48.07 217.3,48.07 217.3,52.45 214.08,55.66 207.37,55.66 205.91,57.12 IC15.3
N$30
  Top 0.381: R53.1 184.29,37.85 184.29,30.54 R51.2
  Bottom 0.381: R51.2 184.29,30.54 186.63,30.54 IC14.2
N$31
  Bottom 0.381: R50.2 184.29,27.92 186.63,27.92 IC14.3
N$32  (via drill 0.35)
  Top 0.381: 200.65,25.29 198.02,27.92 194.51,27.92 IC14.6 | 200.65,25.29 209.41,16.52 IC16.4 | 200.65,25.29 v200.65,29.38
  Bottom 0.381: v200.65,29.38 200.65,34.05 196.85,37.85 R53.2
N$33
  Top 0.381: R54.1 188.09,54.79 188.09,58.29 C59.2
  Bottom 0.381: IC15.2 205.61,59.75 198.31,59.75 VR4.1 198.02,59.46 188.96,59.46 188.09,58.59 C59.2
N$35
  Bottom 0.381: Q3.2 225.48,95.39 227.23,95.39 R57.1 227.52,95.39 233.66,95.39 R55.2
N$36
  Top 0.381: 5B.10 125.87,231.22 125.87,233.55 5B.11 125.58,233.84 122.07,237.35 122.07,266.56 118.28,266.56 5A.7
N$37
  Bottom 0.381: Q4.2 228.1,33.17 232.19,33.17 R58.1 232.49,33.17 238.62,33.17 R56.2
N$38
  Top 0.381: R64.2 222.26,48.07 222.85,47.48 222.85,40.77 Q6.2
  Bottom 0.381: R62.1 221.09,40.77 222.85,40.77 Q6.2
N$39
  Top 0.381: R63.2 221.97,111.75 220.51,110.29 220.51,102.98 Q5.2
  Bottom 0.381: R61.1 218.47,102.98 220.22,102.98 Q5.2
N$40
  Top 0.381: 5A.5 118.28,271.53 122.66,267.14 122.66,239.4 125.58,236.47 5B.12
N$41
  Top 0.381: 5D.4 118.28,167.83 121.78,167.83 121.78,185.36 122.37,185.94 122.37,199.96 125.58,203.18 5C.13
N$42
  Top 0.381: 5E.4 118.28,132.19 121.78,135.7 121.78,163.74 125.58,167.54 5D.13
N$43  (via drill 0.35)
  Top 0.381: v67.45,67.35 67.16,67.64 67.16,86.34 65.7,87.8 63.36,87.8 63.36,88.09 62.78,88.67 v62.78,91.88 | v32.4,111.16 32.4,134.82 26.26,140.96 v24.8,140.96 | v23.05,179.22 v23.05,143.59 | v23.93,181.56 23.93,185.36 32.69,194.12 32.69,210.19 34.44,211.94 34.44,214.57 36.78,216.9 36.78,218.07 34.44,220.41 34.44,250.2 36.78,252.54 36.78,263.06 35.03,264.81 35.03,273.57 36.78,275.32 1A.3
  Bottom 0.381: v67.45,67.35 77.38,67.35 3G.1 | v62.78,91.88 59.56,95.1 40.58,95.1 37.95,97.73 34.73,97.73 31.52,100.94 31.52,110.29 v32.4,111.16 | v24.8,140.96 23.05,142.71 v23.05,143.59 | v23.05,179.22 23.05,180.68 v23.93,181.56
N$44
  Bottom 0.381: IC13.3 149.82,58.59 144.86,58.59 JP4.3
N$45
  Bottom 0.381: IC13.4 149.82,55.96 144.86,55.96 JP4.4
N$46
  Top 0.381: 1E.8 44.37,123.43 42.62,125.18 42.62,131.32 44.37,133.07 1E.12
N$48
  Bottom 0.381: 3H.3 77.67,28.21 81.18,31.71 90.23,31.71 92.86,34.34 108.05,34.34 109.22,35.51 4H.23
N$49  (via drill 0.35)
  Top 0.381: v75.04,15.35 75.04,25.29 76.5,26.75 84.98,26.75 84.98,27.92 3H.14
  Bottom 0.381: v75.04,15.35 62.19,15.35 59.86,17.69 45.83,17.69 44.67,16.52 1H.8
N$50  (via drill 0.35)
  Top 0.381: v86.44,36.68 83.81,36.68 77.67,30.54 3H.2
  Bottom 0.381: v86.44,36.68 110.39,36.68 110.97,36.09 110.97,33.17 109.22,33.17 4H.22
N$51
  Bottom 0.381: 3H.6 77.67,20.32 84.1,26.75 87.9,26.75 92.86,31.71 108.05,31.71 109.22,30.54 4H.21
N$52
  Bottom 0.381: 3H.7 78.26,18.57 81.18,18.57 84.39,21.78 88.19,21.78 93.15,26.75 108.05,26.75 109.22,27.92 4H.20
N$53
  Top 0.381: 1E.6 37.07,125.48 38.82,123.72 38.82,108.24 39.99,107.07 39.99,87.21 39.41,86.63 39.41,81.95 38.82,81.37 38.82,72.31 39.41,71.73 39.41,36.68 35.03,32.3 35.03,28.79 35.9,27.92 41.45,27.92 41.45,22.07 44.37,19.15 1H.9
N$54
  Bottom 0.381: IC13.5 149.82,53.33 144.86,53.33 JP4.5
N$55
  Bottom 0.381: IC13.6 149.82,50.99 144.86,50.99 JP4.6
N$56
  Bottom 0.381: IC13.7 149.82,48.36 144.86,48.36 JP4.7
N$57
  Bottom 0.381: R31.2 191.88,113.21 198.02,113.21 VR1.3
N$58  (via drill 0.35)
  Top 0.381: v62.78,280.58 62.78,248.16 64.53,246.41 2B.19
  Bottom 0.381: v62.78,280.58 57.23,280.58 2A.1
N$59  (via drill 0.35)
  Top 0.381: v60.73,244.07 60.73,271.82 57.23,275.32 2A.3
  Bottom 0.381: v60.73,244.07 64.53,244.07 2B.18
N$60
  Top 0.381: 2B.17 64.53,241.15 61.02,237.64 55.18,237.64 55.18,268.61 56.93,270.36 2A.5
N$61
  Top 0.381: 2B.16 66.57,240.56 66.57,265.98 64.82,267.73 2A.9
N$62
  Top 0.381: 2B.15 64.82,236.47 67.16,238.81 67.16,270.65 64.82,272.99 2A.11
N$63  (via drill 0.35)
  Top 0.381: v68.91,272.11 68.91,237.94 64.82,233.84 2B.14
  Bottom 0.381: v68.91,272.11 67.16,273.86 67.16,277.95 64.82,277.95 2A.13
N$64
  Top 0.381: 2C.1 57.23,209.6 59.27,211.65 59.27,225.08 62.78,228.59 62.78,229.17 64.53,230.92 2B.13
N$65
  Top 0.381: 2C.3 57.23,204.63 59.86,207.26 59.86,223.91 64.53,228.59 2B.12
N$66  (via drill 0.35)
  Top 0.381: v58.98,176.01 58.98,197.62 57.23,199.38 2C.5
  Bottom 0.381: v58.98,176.01 59.56,175.43 64.53,175.43 2D.19
N$67
  Top 0.381: 2D.18 64.82,172.8 66.57,174.55 66.57,195 64.82,196.75 2C.9
N$68  (via drill 0.35)
  Top 0.381: v68.33,201.13 v68.33,170.46
  Bottom 0.381: v68.33,170.46 64.82,170.46 2D.17 | v68.33,201.13 67.74,201.71 64.82,201.71 2C.11
N$69  (via drill 0.35)
  Top 0.381: v68.62,202.3 68.33,202.3 67.45,201.42 67.45,170.46 64.82,167.83 2D.16
  Bottom 0.381: v68.62,202.3 66.57,204.34 66.57,206.97 64.82,206.97 2C.13
N$70
  Top 0.381: 2E.1 57.23,138.62 60.73,142.13 60.73,161.7 63.94,164.91 64.53,164.91 2D.15
N$71
  Bottom 0.381: IC13.8 149.82,45.73 144.86,45.73 JP4.8
N$72  (via drill 0.35)
  Top 0.381: v58.98,139.2 58.98,135.12 57.23,133.36 2E.3 | v58.39,140.96 58.69,141.25 58.69,154.1 58.98,154.39 58.98,157.9 v58.1,158.78
  Bottom 0.381: v58.98,139.2 58.39,139.79 v58.39,140.96 | v58.1,158.78 61.61,162.28 64.53,162.28 2D.14
N$73  (via drill 0.35)
  Top 0.381: v59.86,132.49 59.86,131.03 57.23,128.4 2E.5 | v62.78,157.02 v62.78,135.12
  Bottom 0.381: v59.86,132.49 62.48,135.12 v62.78,135.12 | v62.78,157.02 62.78,159.94 64.53,159.94 2D.13
N$74
  Top 0.381: 2E.9 64.53,125.77 62.78,127.52 62.78,128.69 63.65,129.56 66.57,129.56 67.16,128.98 68.33,128.98 68.33,153.81 64.82,157.31 2D.12
N$75
  Top 0.381: 2G.13 64.82,65.01 66.57,66.76 66.57,84.58 64.82,86.34 2F.12
N$76
  Top 0.381: 2G.11 64.53,59.75 62.78,61.51 62.78,62.67 63.65,63.55 68.33,63.55 68.33,86.04 65.7,88.67 64.82,88.67 2F.13
N$77  (via drill 0.35)
  Top 0.381: v72.12,91.3 72.12,62.09 64.82,54.79 2G.9
  Bottom 0.381: v72.12,91.3 64.82,91.3 2F.14
N$78  (via drill 0.35)
  Top 0.381: v59.86,72.9 59.86,60.05 57.23,57.42 2G.5 | v62.78,72.9 62.78,87.8 61.9,88.67 61.9,92.18 63.65,93.93 64.53,93.93 2F.15
  Bottom 0.381: v62.78,72.9 v59.86,72.9
N$79
  Top 0.381: 5G.4 117.98,61.21 116.23,62.97 116.23,82.25 122.66,88.67 122.66,94.22 124.7,96.27 125.58,96.27 5F.13
N$80
  Top 0.381: 5H.4 118.28,25.29 122.66,25.29 122.66,58 125.58,60.92 5G.13
N$81
  Top 0.381: 9C.2 199.19,208.43 197.43,210.19 197.43,229.17 199.19,230.92 9B.7
N$82
  Top 0.381: 9C.3 199.19,205.8 196.85,208.14 196.85,231.22 199.19,233.55 9B.6
N$83  (via drill 0.35)
  Top 0.381: v195.39,203.47 195.39,240.27 195.97,240.86 197.43,240.86 197.43,238.23 199.19,236.47 9B.5
  Bottom 0.381: v195.39,203.47 199.19,203.47 9C.4
N$84
  Top 0.381: 9B.2 199.48,244.07 201.23,245.82 201.23,264.81 199.48,266.56 9A.7
N$85
  Top 0.381: 9B.3 199.48,241.44 201.82,243.78 201.82,266.85 199.48,269.19 9A.6
N$86
  Top 0.381: 9B.4 199.48,238.81 202.4,241.73 202.4,268.61 199.48,271.53 9A.5
N$87
  Top 0.381: 8C.2 179.03,208.43 177.28,210.19 177.28,229.17 179.03,230.92 8B.7
N$88
  Top 0.381: 8C.3 179.03,205.8 176.69,208.14 176.69,231.22 179.03,233.55 8B.6
N$89
  Top 0.381: 8C.4 179.32,203.47 180.78,204.93 180.78,234.72 179.32,236.18 8B.5
N$90
  Top 0.381: 8B.2 179.32,244.07 180.78,245.53 180.78,265.1 179.32,266.56 8A.7
N$91
  Top 0.381: 8B.3 179.03,241.44 177.28,243.19 177.28,267.44 179.03,269.19 8A.6
N$92
  Top 0.381: 8A.5 181.37,269.48 181.37,240.86 179.32,238.81 8B.4
N$93
  Top 0.381: 2G.3 57.23,62.38 58.98,64.14 58.98,81.08 60.73,82.83 60.73,93.05 63.94,96.27 64.53,96.27 2F.16
N$94  (via drill 0.35)
  Top 0.381: v56.06,82.54 56.06,68.22 56.93,67.35 2G.1 | v71.25,84.87 71.25,92.76 v72.71,94.22
  Bottom 0.381: v56.06,82.54 55.18,83.41 55.18,84.29 55.77,84.87 v71.25,84.87 | v72.71,94.22 67.45,99.48 65.11,99.48 64.82,99.19 2F.17
N$95
  Top 0.381: 2F.18 64.53,101.82 63.07,103.28 61.32,103.28 61.32,132.49 64.53,135.7 2E.13
N$96
  Top 0.381: 2F.19 64.53,104.15 62.78,105.91 62.78,120.22 63.07,120.51 63.07,122.56 62.19,123.43 62.19,128.98 63.94,130.73 64.53,130.73 2E.11
N$97  (via drill 0.35)
  Top 0.381: v75.34,124.89 75.63,124.6 75.63,108.24 81.76,102.11 v81.76,100.94 | v92.28,92.47 87.02,87.21 87.02,56.83 85.85,55.66 83.22,55.66 83.22,53.91 84.98,52.16 3G.8
  Bottom 0.381: v75.34,124.89 71.54,124.89 69.49,126.94 38.24,126.94 37.07,128.11 1E.5 | v81.76,100.94 82.35,100.36 87.02,100.36 92.28,95.1 v92.28,92.47
N$98
  Bottom 0.381: IC13.9 149.82,43.4 144.86,43.4 JP4.9
N$100  (via drill 0.35)
  Top 0.381: v53.72,116.42 v53.72,125.48 | v100.75,116.42 100.75,90.72 100.17,90.13 100.17,81.66 95.2,76.69 95.2,43.1 95.78,42.52 105.13,42.52 105.13,51.87 4G.8
  Bottom 0.381: v53.72,125.48 44.67,125.48 1E.9 | v100.75,116.42 v53.72,116.42
N$101
  Top 0.381: 3E.13 82.64,134.53 82.64,137.45 81.18,138.91 81.18,150.01 81.76,150.6 81.76,166.95 84.98,170.17 3D.14
N$102  (via drill 0.35)
  Top 0.381: v87.61,98.6 87.61,117 81.18,123.43 v81.18,126.35
  Bottom 0.381: v87.61,98.6 87.31,98.6 85.27,96.56 3F.13 | v81.18,126.35 81.18,134.53 84.98,134.53 3E.14
N$105
  Bottom 0.381: IC13.10 149.82,40.77 144.86,40.77 JP4.10
N$106
  Top 0.381: IC13.11 157.42,40.48 155.08,38.14 144.86,38.14 JP4.11
N$107
  Bottom 0.381: IC13.12 157.42,43.1 150.11,35.8 144.86,35.8 JP4.12
N$108
  Bottom 0.381: IC8.1 149.82,124.6 144.86,124.6 JP2.1
N$109
  Bottom 0.381: IC8.2 149.82,121.97 144.86,121.97 JP2.2
N$110
  Bottom 0.381: IC8.3 149.82,119.34 144.86,119.34 JP2.3
N$111
  Top 0.381: 2H.10 64.53,21.78 63.36,22.95 47,22.95 47,25.58 46.42,26.16 44.67,26.16 44.67,26.45 1H.12
N$112  (via drill 0.35)
  Top 0.381: v62.78,30.54 62.78,28.5 64.53,26.75 2H.12
  Bottom 0.381: v62.78,30.54 45.83,30.54 44.67,29.38 1H.13
N$113
  Bottom 0.381: 1H.2 37.07,29.08 38.24,27.92 54.31,27.92 55.47,29.08 56.93,29.08 2H.2
N$114
  Top 0.381: 1H.1 37.07,31.71 40.28,28.5 42.04,28.5 42.04,25.87 43.5,24.41 44.37,24.41 1H.11
N$115
  Top 0.381: R45.1 163.84,45.73 163.84,48.07 R46.1
  Bottom 0.381: IC13.14 157.71,48.07 158.59,47.19 162.67,47.19 163.55,48.07 R46.1
N$116
  Bottom 0.381: C49.1 163.55,50.99 161.21,53.33 157.71,53.33 IC13.16
N$118
  Bottom 0.381: R47.1 161.21,48.36 158.88,50.7 157.71,50.7 IC13.15
N$119
  Bottom 0.381: VR1.1 R30.1
N$120
  Bottom 0.381: C33.1 161.51,114.08 157.71,114.08 IC8.16
N$121
  Top 0.381: R32.1 163.84,106.78 163.84,109.12 R33.1
  Bottom 0.381: IC8.14 157.71,109.12 160.05,106.78 163.55,106.78 R32.1
N$122
  Bottom 0.381: R34.1 161.21,109.41 158.88,111.75 157.71,111.75 IC8.15
N$123
  Bottom 0.381: R10.1 161.21,156.44 160.34,157.31 160.34,163.74 161.21,163.74 LED4.K
N$124
  Bottom 0.381: VR1.2 198.31,110.58 204.44,110.58 C34.1 204.74,110.58 205.91,110.58 213.21,117.88 IC10.5
N$125
  Bottom 0.381: IC8.4 149.82,117 144.86,117 JP2.4
N$126
  Bottom 0.381: R43.1 191.88,45.73 198.02,45.73 VR3.1
N$127
  Bottom 0.381: VR3.2 198.31,48.36 204.44,48.36 C50.1 204.74,48.36 207.07,48.36 213.21,54.5 IC15.5
N$128
  Bottom 0.381: IC8.5 149.82,114.38 144.86,114.38 JP2.5
N$129
  Top 0.381: 3B.13 84.98,238.81 82.35,241.44 82.35,274.15 84.98,276.78 3A.14
N$130
  Bottom 0.381: IC8.6 149.82,111.75 144.86,111.75 JP2.6
N$131
  Bottom 0.381: IC8.7 149.82,109.41 144.86,109.41 JP2.7
N$132
  Bottom 0.381: IC8.8 149.82,106.78 144.86,106.78 JP2.8
N$133
  Bottom 0.381: IC8.9 149.82,104.15 144.86,104.15 JP2.9
N$134
  Bottom 0.381: IC8.10 149.82,101.82 144.86,101.82 JP2.10
N$135
  Top 0.381: IC8.11 157.42,101.52 153.91,98.02 144.86,98.02 144.86,98.9 JP2.11
N$136
  Bottom 0.381: IC8.12 157.42,103.86 152.45,98.9 152.45,96.56 144.86,96.56 JP2.12
N$138
  Bottom 0.381: 6C.8 146.32,194.41 148.95,197.04 156.25,197.04 158.59,199.38 7C.5
N$139  (via drill 0.35)
  Top 0.381: v155.96,204.93 156.25,205.22 156.25,265.39 158.59,267.73 7A.6
  Bottom 0.381: v155.96,204.93 151.57,204.93 146.32,199.67 6C.10
N$140  (via drill 0.35)
  Top 0.381: v156.83,203.47 156.83,261.3 161.21,265.68 v161.21,275.32
  Bottom 0.381: v156.83,203.47 150.99,197.62 146.9,197.62 146.32,197.04 6C.9 | v161.21,275.32 166.18,275.32 7A.12
N$141
  Top 0.381: 7C.10 166.18,199.67 160.63,199.67 159.46,200.84 150.41,200.84 149.53,201.71 146.32,201.71 6C.11
N$155  (via drill 0.35)
  Top 0.381: v88.48,241.15 v88.48,213.11
  Bottom 0.381: v88.48,213.11 75.63,213.11 75.63,207.85 76.5,206.97 80.59,206.97 83.52,204.05 84.39,204.05 84.98,203.47 3C.13 | v88.48,241.15 85.27,241.15 3B.14
N$168
  Top 0.381: 6B.10 146.03,231.22 146.03,233.55 6B.11 146.03,233.84 143.1,236.77 143.1,261.89 138.43,266.56 6A.7
N$169
  Top 0.381: 6A.5 138.43,271.53 143.69,266.27 143.69,238.81 146.03,236.47 6B.12
NINVX
  Top 0.381: IC11.12 215.84,82.83 214.08,84.58 214.08,92.18 221.09,99.19 221.09,102.11 221.97,102.98 221.97,103.86 Q5.1
  Bottom 0.381: R65.1 229.86,106.49 227.52,104.15 222.26,104.15 Q5.1
NINVY
  Top 0.381: IC16.12 217,19.15 215.25,20.9 215.25,29.38 216.13,30.25 216.13,32.3 224.6,40.77 224.6,41.64 Q6.1
  Bottom 0.381: R66.1 234.82,44.27 232.49,41.94 224.89,41.94 Q6.1
P  (via drill 0.35)
  Top 0.381: R3.1 129.67,20.32 130.54,21.2 130.54,32.3 130.84,32.59 130.84,34.05 129.67,35.22 129.67,91.3 R12.1 | 91.69,170.46 96.08,174.84 96.08,197.33 96.95,198.21 99.58,198.21 v99.58,202.88 | 91.69,170.46 89.06,167.83 R5.1 | R13.1 195.68,273.28 199.19,276.78 9A.3 | v89.94,270.07 89.94,274.15 R4.1 | v124.12,263.35 123.83,263.64 123.83,269.77 125.58,271.53 5A.12 | v109.8,266.56 v109.8,200.55 | v120.03,112.33 120.03,100.36 117.11,100.36 116.23,99.48 116.23,98.31 117.98,96.56 5F.4 | v116.81,120.51 v116.81,112.33 | v95.2,167.54 v95.2,131.9 | 91.69,170.46 v91.69,167.54
  Bottom 0.381: 5F.4 118.28,96.27 119.44,95.1 127.91,95.1 129.38,93.64 129.38,91.59 R12.1 | 3D.13 85.27,167.83 88.77,167.83 R5.1 | R6.1 129.38,198.21 128.21,199.38 122.07,199.38 118.28,203.18 5C.4 117.98,203.18 109.8,203.18 | v99.58,202.88 99.87,203.18 109.8,203.18 | 180.49,275.62 179.32,276.78 8A.3 | 180.49,275.62 193.05,275.62 195.39,273.28 R13.1 | 3A.13 85.27,274.45 89.94,274.45 R4.1 | 5A.12 125.87,271.53 126.75,270.65 145.15,270.65 146.03,271.53 6A.12 146.32,271.82 149.82,271.82 R11.1 150.11,271.82 167.35,271.82 171.15,275.62 180.49,275.62 | v89.94,270.07 93.45,266.56 v109.8,266.56 115.94,266.56 117.11,265.39 120.03,265.39 122.07,263.35 v124.12,263.35 | v109.8,200.55 109.8,203.18 | v116.81,112.33 v120.03,112.33 | v116.81,120.51 115.35,121.97 104.25,121.97 102.5,123.72 102.5,131.9 v95.2,131.9 | v91.69,167.54 v95.2,167.54
ROTCLK  (via drill 0.35)
  Top 0.381: 4E.9 105.42,125.48 105.42,123.43 4E.8 105.42,123.14 106.3,122.26 106.3,113.21 | v103.38,63.55 103.67,63.84 103.67,86.04 | 103.67,86.04 105.13,87.5 4F.8 105.42,87.8 105.42,90.13 4F.9 | 106.3,113.21 106.3,106.2 103.67,103.57 103.67,86.04 | 4C.9 105.42,196.75 105.42,194.41 4C.8 105.13,194.12 103.67,192.66 103.67,176.01 | 103.67,176.01 103.67,162.87 105.13,161.4 4D.9 105.42,161.11 105.42,158.78 4D.8 105.42,158.48 105.42,151.76 111.56,145.63 111.56,131.32 111.85,131.03 111.85,114.08 110.97,113.21 106.3,113.21 | 4A.9 105.42,267.73 105.42,265.68 4A.8 105.42,265.39 107.17,263.64 107.17,236.18 104.25,236.18 103.67,235.6 103.67,234.14 105.13,232.68 4B.9 105.42,232.38 105.42,230.05 4B.8 105.13,229.76 105.13,218.07 102.21,215.15 102.21,192.07 101.92,191.78 101.92,176.59 102.5,176.01 103.67,176.01
  Bottom 0.381: v103.38,63.55 96.95,63.55 96.08,62.67 85.56,62.67 85.27,62.38 3G.12
ROTMODE  (via drill 0.35)
  Top 0.381: 96.08,234.14 97.54,232.68 4B.6 | 96.08,234.14 96.08,266.27 97.54,267.73 4A.6 | 4C.6 97.83,196.75 99.58,195 99.58,163.16 97.83,161.4 4D.6 97.54,161.11 96.08,159.65 96.08,137.74 96.66,137.16 99.58,137.16 99.58,134.82 101.62,132.78 v101.62,125.48 101.62,111.16 101.33,110.87 101.33,90.13 v101.04,89.84 101.04,81.66 99.58,80.2 99.58,61.51 97.83,59.75 4G.4 | 96.08,234.14 94.03,232.09 94.03,202.88 93.15,202.01 v93.15,197.04
  Bottom 0.381: v101.04,89.84 100.75,90.13 97.83,90.13 4F.6 | v101.62,125.48 97.83,125.48 4E.6 | v93.15,197.04 97.54,197.04 4C.6
SHCON  (via drill 0.35)
  Top 0.381: IC16.6 209.41,11.56 209.41,13.89 IC16.5 | IC11.6 208.24,74.94 208.24,77.28 IC11.5 | 238.04,52.45 239.79,54.2 239.79,55.66 R28.2 | 238.04,52.45 237.74,52.16 Q2.1 | v235.12,73.77 235.12,59.46 238.04,56.54 238.04,52.45 | 238.04,52.45 Q2.1 | v231.9,12.73 233.66,14.48 233.66,34.92 237.45,38.72 237.45,51.87 Q2.1
  Bottom 0.381: v235.12,73.77 209.41,73.77 208.53,74.65 IC11.6 | v231.9,12.73 210.87,12.73 209.7,11.56 IC16.6
U/DX  (via drill 0.35)
  Top 0.381: 5E.5 117.98,129.56 116.23,131.32 116.23,135.12 117.11,135.99 120.03,135.99 120.03,146.22 120.61,146.8 120.61,162.57 118.28,164.91 5D.5 117.98,165.2 117.4,165.2 115.65,166.95 115.65,173.97 115.06,174.55 115.06,184.77 115.65,185.36 115.65,198.21 117.98,200.55 5C.5 | v169.69,200.55 169.39,200.25 169.39,185.94 168.22,184.77 v168.22,178.05 | v134.34,169.58 v134.34,178.05
  Bottom 0.381: v169.69,200.55 179.03,200.55 8C.5 | v134.34,178.05 v168.22,178.05 | v134.34,169.58 127.33,169.58 126.45,168.71 123.24,168.71 119.74,165.2 118.28,165.2 5D.5
U/DY  (via drill 0.35)
  Top 0.381: v120.03,26.16 120.03,56.54 118.28,58.29 5G.5 | v123.53,93.93 123.24,93.64 123.24,60.63 v121.78,59.17 | v195.39,200.55 195.68,200.25 195.68,178.93 196.56,178.05 196.56,174.55 193.93,171.92 190.13,171.92 190.13,163.16 190.42,162.87 v190.42,159.94 | v151.28,152.35 151.28,145.05 149.82,143.59 149.82,128.69 147.48,126.35 147.48,115.84 v147.19,115.55 | v122.07,114.96 121.49,114.38 121.49,97.43 118.28,94.22 5F.5
  Bottom 0.381: v120.03,26.16 120.03,24.7 118.28,22.95 5H.5 | v123.53,93.93 118.28,93.93 5F.5 | v121.78,59.17 121.2,58.59 118.28,58.59 5G.5 | v195.39,200.55 199.19,200.55 9C.5 | v190.42,159.94 185.46,154.98 163.55,154.98 160.92,152.35 v151.28,152.35 | v147.19,115.55 128.79,115.55 128.21,114.96 v122.07,114.96
UNCONNECTED
  pour Top: 247.65,0 133.35,0 133.35,143.51 129.54,147.32 129.54,151.13 129.54,187.96 247.65,187.96
UNCONNECTED2
  pour Bottom (isolate 0.254): 247.65,0 133.35,0 133.35,64.77 133.35,140.97 128.27,146.05 128.27,177.8 128.27,179.07 128.27,187.96 247.65,187.96
VCC  (via drill 0.35, 0.7, 0.8)
  Top 0.381: R9.2 231.03,204.63 229.27,206.39 229.27,207.56 227.52,209.31 10C.14 | T2.1 132.3,164.91 133.17,164.03 133.17,160.24 R22.2 133.46,159.94 133.46,156.15 | 133.46,156.15 135.8,153.81 R24.2 | v132.59,142.71 132.3,143 132.3,154.98 133.46,156.15
  Top 1.016: 16.51,215.9 17.78,217.17 v35.56,217.17 | 16.51,142.24 v35.56,142.24 | 16.51,109.22 v35.56,109.22 | 16.51,74.93 v35.56,74.93 | 16.51,41.91 v35.56,41.91 | 16.51,180.34 v35.56,180.34 | 16.51,252.73 v35.56,252.73
  Top 2.54: P1.1 4.83,187.96 P1.2 | X3.1 11.99,285.19 16.88,280.3 | 16.51,280.3 16.88,280.3 | 16.88,280.3 17.41,280.3 22.86,285.75 v25.4,285.75
  Top 5.08: 16.51,280.3 16.51,252.73 16.51,215.9 16.51,187.96 | 4.83,187.96 v5.08,187.96 16.51,187.96 | 16.51,187.96 16.51,180.34 16.51,142.24 16.51,109.22 16.51,74.93 16.51,41.91
  Bottom 0.381: v132.59,142.71 125.87,142.71 125.73,142.24
  Bottom 1.016: 9A.16 207.01,285.75 R13.2 186.69,285.75 | 71.12,285.75 44.45,285.75 | 71.12,285.75 90.17,285.75 | 90.17,285.75 105.41,285.75 | 105.41,285.75 125.73,285.75 | 125.73,285.75 146.05,285.75 | 146.05,285.75 149.86,285.75 | 149.86,285.75 166.37,285.75 | 166.37,285.75 186.69,285.75 | 8A.16 186.69,285.75 | R11.2 149.86,285.75 | 90.17,285.75 R4.2 | 1A.14 44.45,285.75 | 3A.5 76.2,271.78 71.12,276.86 71.12,280.67 | 71.12,280.67 71.12,285.75 | 2A.14 71.12,280.67 | 4A.14 105.41,285.75 | 5A.16 125.73,285.75 | 6A.16 146.05,285.75 | 7A.14 166.37,285.75 | 44.45,252.73 71.12,252.73 | 71.12,252.73 105.41,252.73 | 105.41,252.73 125.73,252.73 | 125.73,252.73 146.05,252.73 | 146.05,252.73 166.37,252.73 | 166.37,252.73 186.69,252.73 | 186.69,252.73 207.01,252.73 9B.16 | 8B.16 186.69,252.73 | 7B.14 166.37,252.73 | 6B.16 146.05,252.73 | 5B.16 125.73,252.73 | 4B.14 105.41,252.73 | 3B.5 76.2,236.22 71.12,241.3 71.12,248.92 | 71.12,248.92 71.12,252.73 | 71.12,248.92 2B.20 | 1B.20 44.45,252.73 | 44.45,217.17 C12.1 v35.56,217.17 | 44.45,217.17 C14.1 71.12,217.17 | 71.12,217.17 C16.1 C18.1 105.41,217.17 | 105.41,217.17 C20.1 128.27,217.17 | 128.27,217.17 C22.1 146.05,217.17 | 146.05,217.17 C24.1 166.37,217.17 | 166.37,217.17 C11.1 186.69,217.17 | 186.69,217.17 C13.1 207.01,217.17 | 207.01,217.17 C15.1 227.33,217.17 10C.14 | 9C.16 207.01,217.17 | 186.69,217.17 8C.16 | 7C.14 166.37,217.17 | 6C.14 146.05,217.17 | 5C.16 128.27,210.82 | 128.27,210.82 R6.2 | 128.27,210.82 128.27,217.17 | 4C.14 105.41,217.17 | 3C.5 76.2,200.66 71.12,205.74 71.12,209.55 | 71.12,209.55 71.12,217.17 | 2C.14 71.12,209.55 | 1C.20 44.45,217.17 | 64.77,180.34 44.45,180.34 | 44.45,180.34 v35.56,180.34 | 64.77,180.34 71.12,180.34
  Bottom 1.016: 71.12,180.34 R5.2 105.41,180.34 | 105.41,180.34 125.73,180.34 5D.16 | 4D.14 105.41,180.34 | 3D.5 76.35,166.22 76.22,166.22 71.12,171.32 71.12,180.34 | 2D.20 64.77,180.34 | 5E.16 125.73,142.24 105.41,142.24 | 44.45,142.24 71.12,142.24 | 71.12,142.24 105.41,142.24 | 4E.14 105.41,142.24 | 3E.5 76.2,129.54 71.12,134.62 71.12,138.43 | 71.12,138.43 71.12,142.24 | 2E.14 71.12,138.43 | 1E.14 44.45,142.24 | 105.41,109.22 128.27,109.22 128.27,104.14 | 105.41,109.22 71.12,109.22 | 71.12,109.22 64.77,109.22 | 64.77,109.22 44.45,109.22 | 44.45,109.22 v35.56,109.22 | R12.2 128.27,104.14 | 128.27,104.14 5F.16 | 4F.14 105.41,109.22 | 3F.5 76.35,95.1 76.22,95.1 71.12,100.2 71.12,109.22 | 2F.20 64.77,109.22 | 44.45,74.93 C17.1 v35.56,74.93 | 44.45,74.93 C19.1 64.77,74.93 | 64.77,74.93 C21.1 85.09,74.93 | 85.09,74.93 C23.1 105.41,74.93 | 105.41,74.93 C25.1 125.73,74.93 5G.16 | 4G.14 105.41,74.93 | 3G.14 85.09,74.93 | 2G.14 64.77,74.93 | 1G.20 44.45,74.93 | 109.22,41.91 128.27,41.91 128.27,33.02 | 109.22,41.91 85.09,41.91 | 85.09,41.91 64.77,41.91 | 64.77,41.91 44.45,41.91 | R3.2 128.27,33.02 | 128.27,33.02 5H.16 | 4H.24 109.22,41.91 | 3H.16 85.09,41.91 | 2H.14 64.77,41.91 | 1H.14 44.45,41.91 | v35.56,41.91 44.45,41.91 | 44.45,142.24 v35.56,142.24 | v35.56,252.73 44.45,252.73 | 44.45,285.75 v25.4,285.75 | 1D.20 44.45,180.34 | 1F.20 44.45,109.22
  Bottom 2.54: P1.1 5.08,189.94 v5.08,187.96 5.08,186.49 P1.2
VECTORCOMPLETE  (via drill 0.35)
  Top 0.381: v49.05,134.53 49.34,134.82 49.34,167.25 49.63,167.54 49.63,182.73 v49.34,183.02 | v98.7,192.95 v98.7,183.31
  Bottom 0.381: v49.05,134.53 38.24,134.53 37.07,133.36 1E.3 | v49.34,183.02 83.22,183.02 83.52,183.31 v98.7,183.31 | v98.7,192.95 99,193.24 115.94,193.24 117.11,194.41 133.76,194.41 137.55,198.21 150.41,198.21 156.54,204.34 158.59,204.34 7C.3
VRAM0  (via drill 0.35)
  Top 0.381: P1.3 4.94,182.44 v4.94,183.9 10.49,183.9 11.07,184.48 13.12,184.48 v13.12,153.22 | v40.28,68.81 39.99,69.1 39.99,74.07 39.41,74.65 39.41,81.08 42.04,83.71 42.04,87.5 41.75,87.8 41.75,116.71 v42.04,117 | v33.27,117 33.27,138.33 36.78,141.83 36.78,152.64 35.03,154.39 | v35.03,156.73 35.03,154.39 | v51.97,166.37 v51.97,245.24 | v24.8,153.22 26.26,153.22 30.35,149.14 35.03,149.14 35.03,154.39
  Bottom 0.381: v4.94,183.9 4.94,182.44 P1.3 | v40.28,68.81 37.07,68.81 1G.2 | v33.27,117 v42.04,117 | v35.03,156.73 31.23,160.53 31.23,164.91 36.78,164.91 1D.6 37.07,165.2 38.24,166.37 v51.97,166.37 | v51.97,245.24 37.95,245.24 37.07,246.11 1B.2 | v24.8,153.22 v13.12,153.22
VRAM1  (via drill 0.35)
  Top 0.381: P1.4 4.94,178.05 v4.94,176.59 5.82,175.72 10.49,175.72 v10.49,171.92 | v51.97,67.35 51.68,67.64 51.68,146.51 52.26,147.09 52.26,161.11 v51.97,161.4 | v39.7,161.4 39.99,161.7 39.99,178.64 39.41,179.22 39.41,241.44 37.07,243.78 1B.3 | v24.8,171.92 32.11,171.92 v32.11,163.45
  Bottom 0.381: v4.94,176.59 4.94,178.05 P1.4 | v51.97,67.35 38.24,67.35 37.07,66.18 1G.3 | v51.97,161.4 v39.7,161.4 37.95,161.4 37.07,162.28 1D.7 36.78,162.57 32.98,162.57 v32.11,163.45 | v24.8,171.92 v10.49,171.92
VRAM2  (via drill 0.35)
  Top 0.381: v4.94,172.8 4.94,174.26 P1.5 | v32.4,107.37 v32.4,76.11 | v33.86,111.16 34.15,111.45 v34.15,137.16 | v42.33,137.16 42.33,143.29 43.2,144.17 43.2,152.93 42.62,153.52 42.62,158.78 v42.91,159.07 | v41.45,241.15 41.45,223.04 41.75,222.75 v41.75,189.15 | v37.95,189.15 38.24,188.86 38.24,178.64 38.82,178.05 38.82,164.91 37.66,163.74 35.03,163.74 35.03,161.99 36.78,160.24 1D.8 | v24.8,182.44 32.98,190.61 v32.98,191.78
  Bottom 0.381: v4.94,172.8 4.94,174.26 P1.5 4.94,174.55 7.28,176.89 14,176.89 19.55,182.44 v24.8,182.44 | 1G.4 32.4,67.93 v32.4,76.11 | v32.4,107.37 33.86,108.83 v33.86,111.16 | v42.33,137.16 v34.15,137.16 | v42.91,159.07 42.04,159.94 37.07,159.94 1D.8 | v41.45,241.15 37.07,241.15 1B.4 | v37.95,189.15 38.82,189.15 | 38.82,189.15 v41.75,189.15 | v32.98,191.78 37.95,191.78 38.82,190.91 38.82,189.15
VRAM3  (via drill 0.35)
  Top 0.381: v4.36,171.92 4.65,171.63 4.65,170.46 P1.6 4.94,170.17 7.28,167.83 10.49,167.83 v10.49,157.61 | v80.01,65.89 80.01,90.72 80.89,91.59 v80.89,94.81 | v74.46,125.77 v74.46,98.6 | v67.45,153.52 v67.45,129.86 | 1B.5 38.82,236.77 38.82,178.93 39.41,178.35 39.41,162.28 38.82,161.7 38.82,159.36 37.07,157.61 1D.9 36.78,157.61 v24.8,157.61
